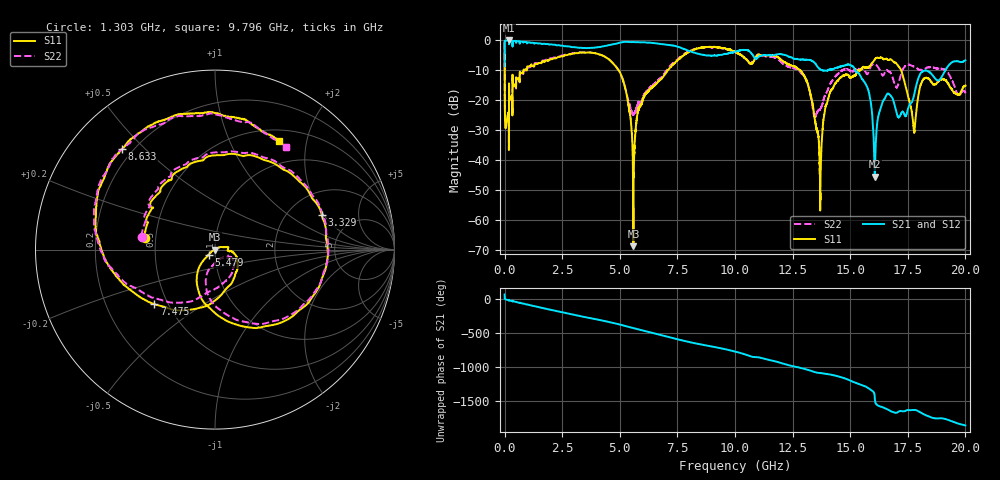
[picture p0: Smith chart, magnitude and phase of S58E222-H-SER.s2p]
!{S58E222}
!Johanson Technology Inc.
!www.johansontechnology.com
!Test Board Conditions:
!Substrate Type  RO4350B
!Substrate Thickness  60 mil
!Substrate Dk  3.66
!TL Type: GCPW
!TL Trace Width  115 mil
!TL Gap  52 mil
!Electrode orientation  Horizontal
!DUT TOPOLOGY	SERIES
!Mounting Pad LxW  55x428 mil
! Created Wed Apr 14 11:32:30 2021
# mhz S ma R 50
! 2 Port Network Data from SP1.SP block
! freq  magS11  angS11  magS21  angS21  magS12  angS12  magS22  angS22
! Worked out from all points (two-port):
!   20001 points, 300 kHz to 20 GHz, reference 50 ohm
!   highest |S21| = -0.02 dB at 185.3 MHz (marker M1); lowest = -45.6 dB at 16.07 GHz (marker M2)
!   |S21| within 3 dB of the highest: 1.064 MHz to 7.855 GHz (7.853 GHz wide, 200 % of centre)
!   lowest |S11| = -68.7 dB at 5.589 GHz (marker M3), VSWR 1.00, Z = 50 + j0.0269 ohm
!   |S11| at or under -10 dB: 4.951 GHz to 7.078 GHz (2.127 GHz wide, 35.4 % of centre); 12.83 GHz to 15.34 GHz (2.502 GHz wide, 17.8 % of centre); 17.21 GHz to end of sweep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
!   |S22| runs from -36.5 to -0.7 dB; largest |S21 - S12| = 0.0059
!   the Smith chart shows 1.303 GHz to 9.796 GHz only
!   S11 on the Smith chart (normalised r, x): 1.303 GHz: 0.43, +0.07; 3.329 GHz: 3.04, +1.91; 5.479 GHz: 0.93, -0.05; 7.475 GHz: 0.42, -0.32; 8.633 GHz: 0.16, +0.43; 9.796 GHz: 0.66, +1.56
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0.3  0.9247 -22.1  0.3716 67.7  0.3699 67.7  0.9253 -22.0
185.3  0.03569 -110.1  0.9983 -17.8  0.9986 -17.7  0.03398 -106.8
1303.3  0.397 170.3  0.8887 -103.4  0.8873 -103.4  0.4142 169.9
3329.3  0.6252 17.8  0.7527 107.2  0.7533 107.1  0.6306 19.4
3334.3  0.6247 17.5  0.7526 106.8  0.7522 106.8  0.6307 19.1
4917.3  0.3277 -94.9  0.895 -6.3  0.8938 -6.4  0.3327 -86.1
5479.3  0.04559 -140.2  0.936 -55.8  0.9378 -55.8  0.07149 -87.8
5589.3  0.0003657 47.2  0.9387 -65.3  0.9365 -65.2  0.05862 -61.6
6667.3  0.2054 -62.2  0.8853 -157.8  0.8838 -157.9  0.2165 -88.2
7475.3  0.4544 -138.1  0.7935 133.1  0.7931 133.1  0.4698 -149.7
8633.3  0.7628 132.8  0.5741 47.1  0.5721 47.2  0.7639 136.7
9796.3  0.7015 59.3  0.6237 -32.5  0.6251 -32.5  0.6959 55.3
10000.3  0.6465 42.7  0.6489 -49.0  0.6504 -49.0  0.6371 39.1
11547.3  0.5639 -74.4  0.565 -178.5  0.5641 -178.6  0.5337 -76.0
13334.3  0.1015 165.7  0.4576 23.0  0.4585 22.9  0.09031 172.0
13697.3  0.001439 -105.6  0.3283 -5.8  0.3275 -5.7  0.07168 -108.7
14158.3  0.145 -67.1  0.3276 -29.1  0.3249 -29.2  0.1957 -104.1
15391.3  0.3124 162.4  0.2753 -167.3  0.2723 -167.6  0.3335 130.5
16067.3  0.4814 106.8  0.005274 -10.4  0.005348 -9.4  0.4077 82.5
16667.3  0.4705 50.9  0.1287 172.2  0.1262 171.7  0.3047 55.4
17764.3  0.03134 -109.2  0.1179 173.6  0.1184 174.0  0.366 8.6
20000  0.1757 -102.1  0.4654 -55.9  0.4661 -55.8  0.134 179.5
